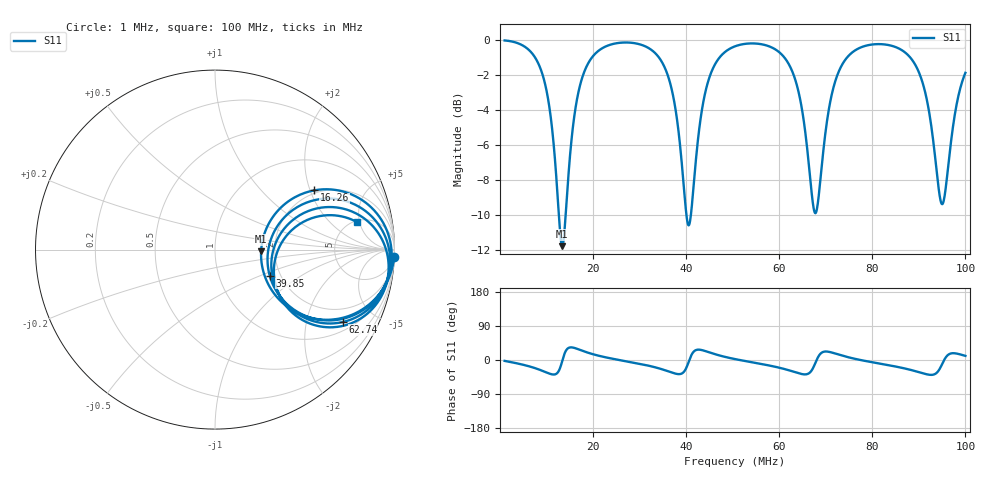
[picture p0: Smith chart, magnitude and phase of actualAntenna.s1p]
# MHz S RI R 50.0
! SimSmith 18.4g
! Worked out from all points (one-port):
!   1000 points, 1 MHz to 100 MHz, reference 50 ohm
!   lowest |S11| = -11.8 dB at 13.39 MHz (marker M1), VSWR 1.69, Z = 84.5 - j1.86 ohm
!   |S11| at or under -10 dB: 12.66 MHz to 14.12 MHz (1.464 MHz wide, 10.9 % of centre); 40.06 MHz to 41.03 MHz (966.5 kHz wide, 2.38 % of centre)
!   S11 on the Smith chart (normalised r, x): 1 MHz: 1, -49; 16.26 MHz: 1.89, +2.13; 39.85 MHz: 1.76, -0.57; 62.74 MHz: 1.34, -3.28; 100 MHz: 5.25, +4.60
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1  0.998 -0.0403
6.351351  0.8939 -0.2728
9.918919  0.6126 -0.391
11.6036  0.3866 -0.3055
13.38739  0.2569 -0.0103
16.26126  0.5522 0.3299
20.12613  0.8751 0.2306
25.77478  0.9836 -0.00568
33.20721  0.8733 -0.2978
38.16216  0.4604 -0.3477
39.84685  0.3047 -0.1446
40.93694  0.3064 0.0412
43.51351  0.5814 0.2807
46.58559  0.8446 0.2101
50.54955  0.9608 0.0384
57.68469  0.9335 -0.2344
62.73874  0.7119 -0.4036
62.93694  0.696 -0.4068
65.41441  0.4491 -0.3506
67.69369  0.3153 -0.0543
70.66667  0.5899 0.2336
75.32432  0.9097 0.092
81.66667  0.9613 -0.1628
87.71171  0.8246 -0.3754
91.67568  0.5378 -0.4154
94.54955  0.3282 -0.1316
97.12613  0.5139 0.1652
100  0.7924 0.1526
